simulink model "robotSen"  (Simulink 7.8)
settings: Solver=ode3  StartTime=0.0  StopTime=15  FixedStep=0.1  RelTol=1e-3
InitFcn:
  | M=csvread('map1.csv');
  | assignin('base','M',M);
  | SensorOrients=[80 50 25 0 -25 -50 -80 130 -130];
  | assignin('base','SensorOrients',SensorOrients);
  | SensorAngle=20;
  | assignin('base','SensorAngle',SensorAngle);
  | SensorRange=0.6;
  | assignin('base','SensorRange',SensorRange);
  | prevGD=inf;
  | assignin('base', 'prevGD', prevGD);
undefined symbols (not defined in the file or in its folder): controlRobot, simRobotMdl
libraries: simulink x1

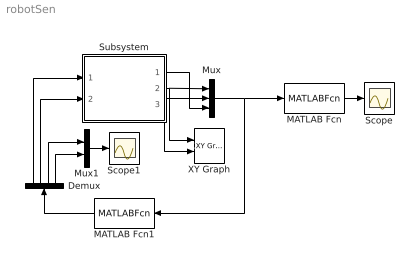
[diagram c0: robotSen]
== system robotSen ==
  Demux : Demux
  MATLAB Fcn : MATLABFcn  MATLABFcn=simRobotMdl(u(1),u(2),u(3))
  MATLAB Fcn1 : MATLABFcn  MATLABFcn=controlRobot(u(1),u(2),u(3))
  Mux : Mux  Inputs=3
  Mux1 : Mux  Inputs=2
  Scope : Scope
  Scope1 : Scope
  Subsystem : Subsystem
  XY Graph : simulink/Sinks/XY Graph  xmin=-1  xmax=2  ymin=-1  ymax=2  st=-1
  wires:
  Demux/1 -> Subsystem/1(Omeaga L)
  Demux/2 -> Subsystem/2(Omega R)
  Subsystem/2(X) -> Mux/1, XY Graph/1
  Subsystem/3(Y) -> Mux/2, XY Graph/2
  Subsystem/1(Theta) -> Mux/3
  Mux/1 -> MATLAB Fcn/1, MATLAB Fcn1/1
  MATLAB Fcn/1 -> Scope/1
  MATLAB Fcn1/1 -> Demux/1
  Mux1/1 -> Scope1/1
  Demux/3 -> Mux1/1
  Demux/4 -> Mux1/2

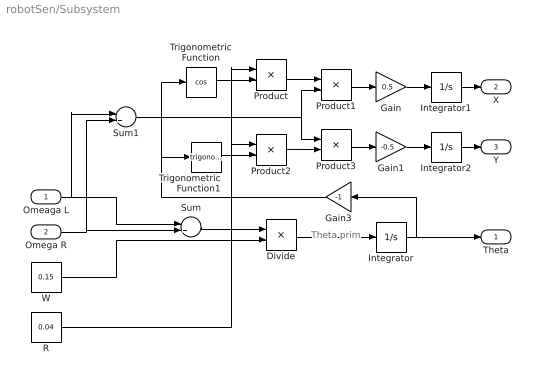
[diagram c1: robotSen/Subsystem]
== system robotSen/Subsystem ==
  note: Theta prim
  Omeaga L : Inport
  Omega R : Inport  Port=2
  Divide : Product  Inputs=*/
  Gain : Gain  Gain=0.5
  Gain1 : Gain  Gain=-0.5
  Gain3 : Gain  Gain=-1
  Integrator : Integrator
  Integrator1 : Integrator
  Integrator2 : Integrator
  Product{,1..3} (4 alike) : Product
  R : Constant  Value=0.04
  Sum : Sum  Inputs=-+
  Sum1 : Sum
  Trigonometric Function : Trigonometry  Operator=cos
  Trigonometric Function1 : Trigonometry
  W : Constant  Value=0.15
  Theta : Outport
  X : Outport  Port=2
  Y : Outport  Port=3
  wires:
  Omeaga L/1 -> Sum/1, Sum1/1
  Omega R/1 -> Sum/2, Sum1/2
  Sum/1 -> Divide/1
  W/1 -> Divide/2
  Divide/1 -> Integrator/1
  Integrator/1 -> Gain3/1, Theta/1
  Trigonometric Function/1 -> Product/2
  Product/1 -> Product1/1
  Sum1/1 -> Product1/2, Product3/1
  Product1/1 -> Gain/1
  Gain/1 -> Integrator1/1
  Product3/1 -> Gain1/1
  Gain1/1 -> Integrator2/1
  Trigonometric Function1/1 -> Product2/2
  Integrator1/1 -> X/1
  Integrator2/1 -> Y/1
  Product2/1 -> Product3/2
  R/1 -> Product/1, Product2/1
  Gain3/1 -> Trigonometric Function/1, Trigonometric Function1/1
